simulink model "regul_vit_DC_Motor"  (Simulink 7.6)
settings: Solver=ode15s  StartTime=0.0  StopTime=200  RelTol=1e-3
InitFcn:
  | clear all
  | close all
  | Kp=0.005;
  | Ti=0.5;
StopFcn:
  | load pos_vit.mat
  | plot(x(1,:),x(3,:), x(1,:),x(5,:))
  | grid
  | title('Consigne et vitesse mesurée')
  | xlabel('temps')
  | 
  | figure
  | plotyy(x(1,:),x(2,:), x(1,:),x(4,:))
  | grid
  | title('Signal de commande et déplacement linéaire x')
  | xlabel('temps')
libraries: fl_lib x17, nesl_utility x5, elec_lib x1

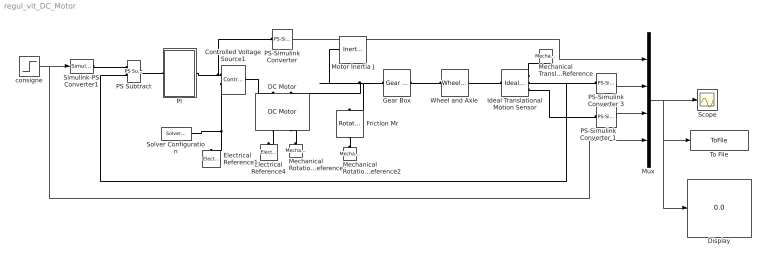
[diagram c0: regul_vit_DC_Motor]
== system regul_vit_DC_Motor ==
  Controlled Voltage Source1 : fl_lib/Electrical/Electrical Sources/Controlled Voltage Source  DialogController=NetworkEngine.DynNeDlgSource  SystemSampleTime=-1  i_Log=off  v_Log=off  LocalVarNames=|current|voltage|power  LocalVarDescs=|Current (A)|Voltage (V)|Power (W)  LocalVarLogging=[0 0 0]
  DC Motor : elec_lib/Actuators & Drivers/Rotational Actuators/DC Motor  DialogController=NetworkEngine.DynNeDlgSource  SystemSampleTime=-1  parameterization=1  Ra=3.9 Ohm  La=1.2e-05 H  emf_or_torque=1  Kv=7.2e-05 V/rpm  Ki=6.876e-04 N*m/A  T_stall=2.4e-04 N*m  w_max=1.91e+04 rpm  w_rated=1.5e+04 rpm  P_rated=0.08 W  V_rated=1.5 V  J=0.01 g*cm^2  lam=1e-08 N*m/(rad/s)  speed0=0 rpm  current_Log=off  voltage_Log=off  power_Log=off  i2r_Log=off  torque_Log=off  speed_Log=off  LocalVarNames=|current|voltage|power|i2r|torque|speed  LocalVarDescs=|Current (A)|Voltage (V)|Power (W)|Electrical losses (W)|Torque (Nm)|Angular speed (rad/s)  LocalVarLogging=[0 0 0 0 0 0]
  Display : Display
  Electrical Reference1 : fl_lib/Electrical/Electrical Elements/Electrical Reference  DialogController=NetworkEngine.DynNeDlgSource  SystemSampleTime=-1  i_Log=off  LocalVarNames=|i  LocalVarDescs=|i  LocalVarLogging=[]
  Electrical Reference4 : fl_lib/Electrical/Electrical Elements/Electrical Reference  DialogController=NetworkEngine.DynNeDlgSource  SystemSampleTime=-1  i_Log=off  LocalVarNames=|i  LocalVarDescs=|i  LocalVarLogging=[]
  Friction Mr : fl_lib/Mechanical/Rotational Elements/Rotational Friction  DialogController=NetworkEngine.DynNeDlgSource  SystemSampleTime=-1  brkwy_trq=0.02e-3 N*m  Col_trq=0.02e-3 N*m  visc_coef=0 N*m/(rad/s)  trans_coef=10 s/rad  vel_thr=0.1 rad/s  t_Log=off  w_Log=off  LocalVarNames=|friction_torque|rel_velocity|power  LocalVarDescs=|Friction torque (N*m)|Relative velocity (rad/s)|Power (W)  LocalVarLogging=[0 0 0]
  Gear Box : fl_lib/Mechanical/Mechanisms/Gear Box  DialogController=NetworkEngine.DynNeDlgSource  SystemSampleTime=-1  ratio=5  t_in_Log=off  t_out_Log=off  LocalVarNames=|t_in|t_out  LocalVarDescs=|t_in|t_out  LocalVarLogging=[0 0]
  Ideal Translational Motion Sensor : fl_lib/Mechanical/Mechanical Sensors/Ideal Translational Motion Sensor  DialogController=NetworkEngine.DynNeDlgSource  SystemSampleTime=-1  offset=0 m  v_Log=off  f_Log=off  x_Log=off  LocalVarNames=|v|f|x  LocalVarDescs=|v|f|x  LocalVarLogging=[0 0 0]
  Mechanical Rotational Reference1 : fl_lib/Mechanical/Rotational Elements/Mechanical Rotational Reference  DialogController=NetworkEngine.DynNeDlgSource  SystemSampleTime=-1  t_Log=off  LocalVarNames=|t  LocalVarDescs=|t  LocalVarLogging=[]
  Mechanical Rotational Reference2 : fl_lib/Mechanical/Rotational Elements/Mechanical Rotational Reference  DialogController=NetworkEngine.DynNeDlgSource  SystemSampleTime=-1  t_Log=off  LocalVarNames=|t  LocalVarDescs=|t  LocalVarLogging=[]
  Mechanical Translational Reference : fl_lib/Mechanical/Translational Elements/Mechanical Translational Reference  DialogController=NetworkEngine.DynNeDlgSource  SystemSampleTime=-1  f_Log=off  LocalVarNames=|f  LocalVarDescs=|f  LocalVarLogging=0
  Motor Inertia J : fl_lib/Mechanical/Rotational Elements/Inertia  DialogController=NetworkEngine.DynNeDlgSource  SystemSampleTime=-1  inertia=10 g*cm^2  initial_velocity=0 rad/s  t_Log=off  LocalVarNames=|torque|velocity  LocalVarDescs=|Inertia torque (N*m)|Inertia absolute velocity (rad/s)  LocalVarLogging=[0 0]
  Mux : Mux
  PI : Subsystem
  PS Subtract : fl_lib/Physical Signals/Functions/PS Subtract  DialogController=NetworkEngine.DynNeDlgSource  SystemSampleTime=-1  LocalVarLogging=[]
  PS-Simulink Converter : nesl_utility/PS-Simulink Converter  DialogController=NetworkEngine.DynNeUtilDlgSource  SystemSampleTime=-1  PhysicalDomain=network_engine_domain  LeftPortType=input  RightPortType=output  SubClassName=ps_output  Unit=1  AffineConversion=off
  PS-Simulink Converter 1 : nesl_utility/PS-Simulink Converter  DialogController=NetworkEngine.DynNeUtilDlgSource  SystemSampleTime=-1  PhysicalDomain=network_engine_domain  LeftPortType=input  RightPortType=output  SubClassName=ps_output  Unit=1  AffineConversion=off
  PS-Simulink Converter 3 : nesl_utility/PS-Simulink Converter  DialogController=NetworkEngine.DynNeUtilDlgSource  SystemSampleTime=-1  PhysicalDomain=network_engine_domain  LeftPortType=input  RightPortType=output  SubClassName=ps_output  Unit=1  AffineConversion=off
  Scope : Scope
  Simulink-PS Converter1 : nesl_utility/Simulink-PS Converter  DialogController=NetworkEngine.DynNeUtilDlgSource  SystemSampleTime=-1  PhysicalDomain=network_engine_domain  LeftPortType=input  RightPortType=output  SubClassName=ps_input  Unit=1  AffineConversion=off  InputFilterTimeConstant=.001  UdotUserProvided=0
  Solver Configuration : nesl_utility/Solver Configuration  DialogController=NetworkEngine.DynNeUtilDlgSource  SystemSampleTime=-1  PhysicalDomain=network_engine_domain  LeftPortType=input  RightPortType=generic  SubClassName=solver  Accelerate=off  Profile=off  ResidualTolerance=1e-9  MaxNonlinIter=12  MaxModeIter=2  DoFixedCost=off  UseLocalSampling=off  DoDC=off  LinearAlgebra=Full  LocalSolverSampleTime=.001  LocalSolverChoice=NE_BACKWARD_EULER_ADVANCER  UseLocalSolver=off
  To File : ToFile  Filename=pos_vit.mat  MatrixName=x
  Wheel and Axle : fl_lib/Mechanical/Mechanisms/Wheel and Axle  DialogController=NetworkEngine.DynNeDlgSource  SystemSampleTime=-1  R=0.05 m  or=1  torque_A_Log=off  force_P_Log=off  ang_velocity_Log=off  velocity_Log=off  LocalVarNames=|torque_A|force_P|ang_velocity|velocity  LocalVarDescs=|Axle torque (N*m)|Periphery force (N)|Axle angular velocity (rad/s)|Periphery velocity (m/s)  LocalVarLogging=[0 0 0 0]
  consigne : Step  Time=10  After=0.5  SampleTime=0
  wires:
  Mux/1 -> Scope/1, To File/1, Display/1
  consigne/1 -> Simulink-PS Converter1/1, Mux/4
  PS-Simulink Converter 3/1 -> Mux/2
  PS-Simulink Converter 1/1 -> Mux/3
  PS-Simulink Converter/1 -> Mux/1
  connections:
  Ideal Translational Motion Sensor/RConn1 -- Mechanical Translational Reference/LConn1
  Simulink-PS Converter1/RConn1 -- PS Subtract/LConn1
  Mechanical Rotational Reference1/LConn1 -- DC Motor/RConn2
  Gear Box/LConn1 -- Motor Inertia J/LConn1 -- DC Motor/LConn2 -- Friction Mr/LConn1
  Wheel and Axle/LConn1 -- Gear Box/RConn1
  Wheel and Axle/RConn1 -- Ideal Translational Motion Sensor/LConn1
  Friction Mr/RConn1 -- Mechanical Rotational Reference2/LConn1
  DC Motor/RConn1 -- Electrical Reference4/LConn1
  Controlled Voltage Source1/LConn1 -- DC Motor/LConn1
  Controlled Voltage Source1/RConn2 -- Electrical Reference1/LConn1 -- Solver Configuration/RConn1
  Controlled Voltage Source1/RConn1 -- PS-Simulink Converter/LConn1 -- PI/RConn1
  Ideal Translational Motion Sensor/RConn2 -- PS-Simulink Converter 3/LConn1 -- PS Subtract/LConn2
  Ideal Translational Motion Sensor/RConn3 -- PS-Simulink Converter 1/LConn1
  PS Subtract/RConn1 -- PI/LConn1

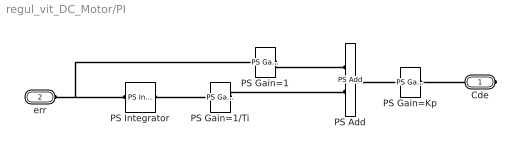
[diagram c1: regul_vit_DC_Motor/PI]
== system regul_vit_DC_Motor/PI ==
  PS Add : fl_lib/Physical Signals/Functions/PS Add  DialogController=NetworkEngine.DynNeDlgSource  SystemSampleTime=-1  LocalVarLogging=[]
  PS Gain=1 : fl_lib/Physical Signals/Functions/PS Gain  DialogController=NetworkEngine.DynNeDlgSource  SystemSampleTime=-1  gain=1  LocalVarLogging=[]
  PS Gain=1/Ti : fl_lib/Physical Signals/Functions/PS Gain  DialogController=NetworkEngine.DynNeDlgSource  SystemSampleTime=-1  gain=1/Ti  LocalVarLogging=[]
  PS Gain=Kp : fl_lib/Physical Signals/Functions/PS Gain  DialogController=NetworkEngine.DynNeDlgSource  SystemSampleTime=-1  gain=Kp  LocalVarLogging=[]
  PS Integrator : fl_lib/Physical Signals/Linear Operators/PS Integrator  DialogController=NetworkEngine.DynNeDlgSource  SystemSampleTime=-1  x0=0  x_Log=off  LocalVarNames=|x  LocalVarDescs=|x  LocalVarLogging=0
  Cde : PMIOPort  Port=1  Side=Right
  err : PMIOPort  Port=2  Side=Left
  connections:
  PS Gain=1/RConn1 -- PS Add/LConn1
  PS Gain=1/Ti/RConn1 -- PS Add/LConn2
  PS Add/RConn1 -- PS Gain=Kp/LConn1
  PS Integrator/RConn1 -- PS Gain=1/Ti/LConn1
  Cde/RConn1 -- PS Gain=Kp/RConn1
  err/RConn1 -- PS Integrator/LConn1 -- PS Gain=1/LConn1
